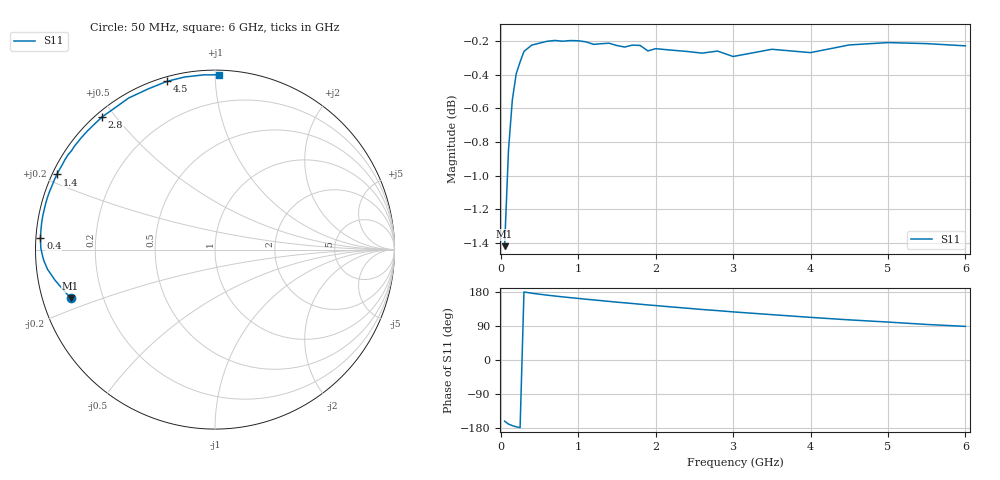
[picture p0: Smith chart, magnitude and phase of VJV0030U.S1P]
! Infineon Technologies  Discrete & RF Semiconductors
! BB 914
! Si Tuning Diode in SOT23
! VR =
! S-Parameters:  July  1999
# GHz  S  MA  R  50
!  f  S11
! GHz  MAG  ANG
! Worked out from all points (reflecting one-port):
!   34 points, 50 MHz to 6 GHz, reference 50 ohm
!   lowest |S11| = -1.4 dB at 50 MHz (marker M1), VSWR 12.26, Z = 4.19 - j8.13 ohm
!   phase of S11 starts at -161 deg and turns -110 deg over the sweep
!   S11 on the Smith chart (normalised r, x): 50 MHz: 0.08, -0.16; 400 MHz: 0.01, +0.03; 1.4 GHz: 0.01, +0.23; 2.8 GHz: 0.02, +0.46; 4.5 GHz: 0.02, +0.75; 6 GHz: 0.03, +1.02
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0.05  0.8491 -161.4
0.1  0.9069 -169.1
0.15  0.9388 -173.2
0.2  0.9558 -176.3
0.25  0.9635 -178.5
0.3  0.9704 179.5
0.4  0.9747 176.3
0.6  0.9772 171.1
0.8  0.9773 166.6
1  0.9776 162.5
1.1  0.9769 160.4
1.4  0.9759 154.6
1.5  0.9744 152.6
1.6  0.9734 150.9
1.8  0.9744 147.2
1.9  0.9708 145.3
2  0.9723 143.7
2.2  0.9713 140.1
2.4  0.9705 136.8
2.6  0.9693 133.3
2.8  0.9707 130.3
3  0.9671 127.0
3.5  0.9719 119.7
4  0.9697 112.5
4.5  0.9748 105.9
5  0.9764 100.1
5.5  0.9757 93.8
6  0.9742 88.7
